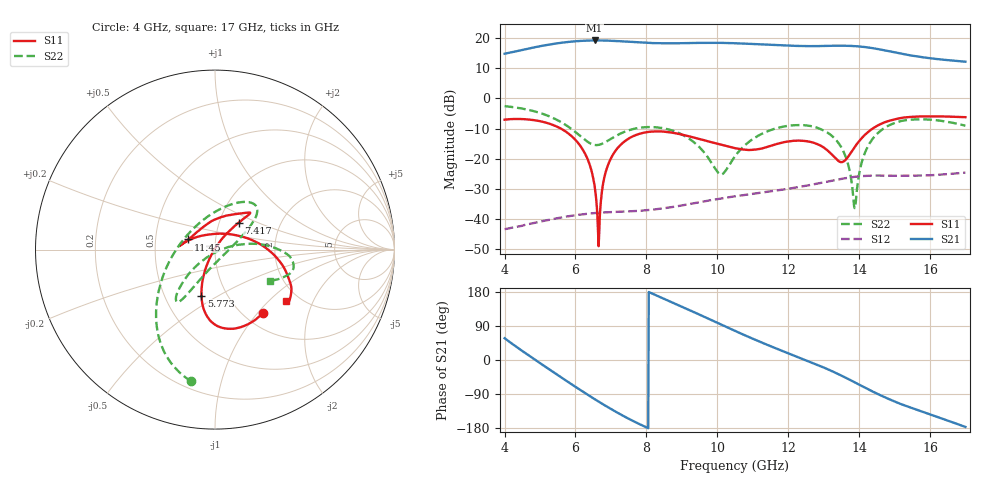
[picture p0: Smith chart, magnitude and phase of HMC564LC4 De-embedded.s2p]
! Hittite Microwave Corporation
! 20 Alpha Road
! Chelmsford, MA 01824
! http://www.hittite.com
! Tel: 978-250-3343
! Fax: 978-250-3373
! Device:  HMC564LC4
! Description: GaAs SMT PHEMT LOW NOISE amplifier
! Frequency:  7 - 14 GHz
! Package:  LC4  - RoHS Compliant 4*4  package - 24 pins
! Ports:  2
! Voltages:  V1 =+3.0 Volts
!  v2 =+3  Volts
! Data:  The device was measured on evaluation board 116156.
!  The evaluation circuit board was modeled and simulated.  This was use
!  to removed the evaluation board circuit from the measured data.
!  The reference plane is the center of the package pin.
! Misc:
! Date Measured:  28-11-2007
! Date:  29-11-2007
! Note:
!  Hittite Microwave supplies this data as a sample of measured data at the
!  package pin for this package product.  Your particular data for this product
!  may vary.
!  Data was taken at 25 degrees C.
!  Hittite Microwave reserves the right to change this data at anytime.
# MHz S MA R 50
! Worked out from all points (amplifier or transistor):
!   800 points, 4 GHz to 17 GHz, reference 50 ohm
!   highest |S21| = 19.2 dB at 6.538 GHz (marker M1)
!   |S21| within 3 dB of that: 4.553 GHz to 14.6 GHz (10.04 GHz wide, 105 % of centre)
!   unconditionally stable (mu >= 1): start of sweep to end of sweep
!   at 6.164 GHz: K = 4.40, MAG = 19.4 dB, |S12| = -38.5 dB
!   at 10.51 GHz: K = 2.56, MAG = 18.5 dB, |S12| = -32.5 dB
!   at 17 GHz: K = 1.41, MAG = 14.6 dB, |S12| = -24.6 dB
!   S11 on the Smith chart (normalised r, x): 4 GHz: 1.21, -1.07; 5.773 GHz: 0.76, -0.42; 7.417 GHz: 1.24, +0.39; 11.45 GHz: 0.74, +0.09; 17 GHz: 1.70, -1.28
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4000  0.4432 -53.2  5.506 57.5  0.006768 142.1  0.7447 -100.4
4471.84  0.4541 -74.6  6.313 25.6  0.007642 123.0  0.6811 -110.7
4976.22  0.4209 -89.4  7.295 -6.8  0.008969 105.5  0.5786 -122.8
5366.71  0.3616 -98.3  7.996 -31.5  0.009925 92.3  0.4727 -133.9
5773.47  0.2685 -106.3  8.609 -56.9  0.01102 78.7  0.346 -149.7
6180.23  0.1491 -114.2  9.004 -81.8  0.01186 65.3  0.2257 -176.4
6538.17  0.03549 -124.5  9.137 -103.2  0.01252 54.2  0.1685 141.2
6668.34  0.005741 92.8  9.133 -110.7  0.01269 50.3  0.1699 123.4
6993.74  0.09962 54.4  9.032 -128.9  0.01293 40.9  0.212 89.1
7416.77  0.1994 48.7  8.751 -150.9  0.01326 30.8  0.2839 66.0
8344.18  0.2837 46.5  8.215 167.8  0.01465 13.3  0.3277 44.3
8962.45  0.2536 52.9  8.227 142.4  0.01659 2.5  0.2584 35.8
9580.73  0.2059 68.6  8.341 116.1  0.01925 -9.8  0.137 21.4
10508.1  0.1489 106.6  8.213 76.4  0.02373 -31.2  0.1109 -105.1
11451.8  0.1594 159.2  7.741 38.4  0.02829 -52.3  0.2892 -121.8
12672.1  0.1869 170.9  7.357 -7.0  0.03708 -79.1  0.3439 -129.2
13322.9  0.1031 130.0  7.466 -33.2  0.04402 -96.4  0.2126 -136.5
13924.9  0.1707 24.6  7.332 -61.2  0.05037 -116.8  0.02483 -9.6
14331.7  0.3001 -0.7  6.887 -80.8  0.0523 -131.5  0.1929 9.6
14836  0.4221 -18.5  6.079 -102.9  0.05199 -147.7  0.3541 0.1
15779.7  0.5023 -34.0  4.82 -136.4  0.05243 -171.7  0.4494 -13.8
17000  0.4875 -36.0  4.06 -176.6  0.05866 159.1  0.3523 -29.9
